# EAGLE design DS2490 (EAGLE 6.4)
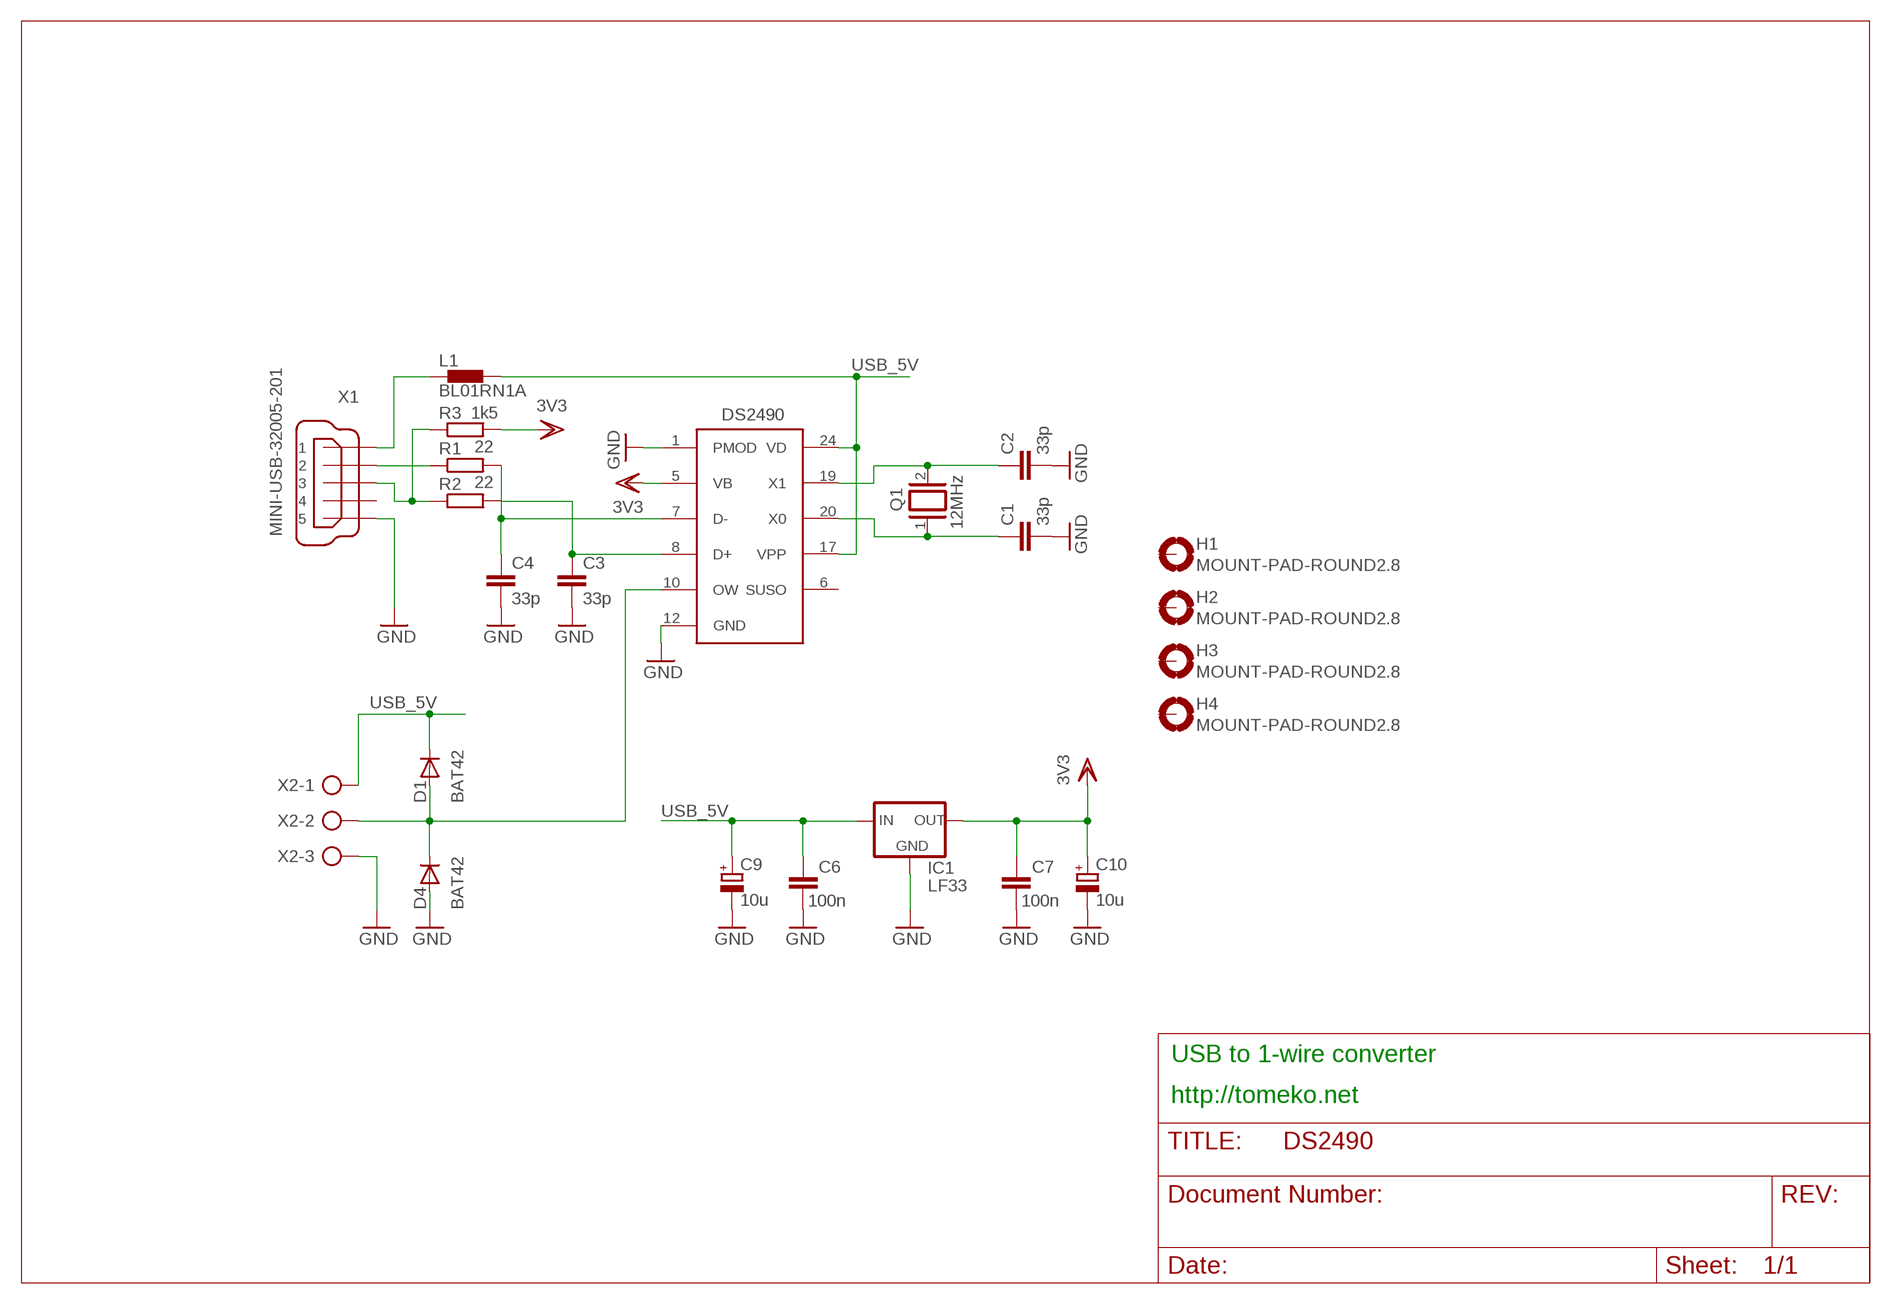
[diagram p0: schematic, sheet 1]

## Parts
C1  33p  C-EUC0805K  [C0805K]
C2  33p  C-EUC0805K  [C0805K]
C3  33p  C-EUC0805K  [C0805K]
C4  33p  C-EUC0805K  [C0805K]
C6  100n  C-EUC0805K  [C0805K]
C7  100n  C-EUC0805K  [C0805K]
C9  10u  CPOL-EUCT3216  [CT3216]
C10  10u  CPOL-EUCT3216  [CT3216]
D1  BAT42  1N4148DO35-7  [DO35-7]
D4  BAT42  1N4148DO35-7  [DO35-7]
H1  MOUNT-PAD-ROUND2.8  [2,8-PAD]
H2  MOUNT-PAD-ROUND2.8  [2,8-PAD]
H3  MOUNT-PAD-ROUND2.8  [2,8-PAD]
H4  MOUNT-PAD-ROUND2.8  [2,8-PAD]
IC1  LF33  LFXXCV  [DPACK_1]
L1  BL01RN1A  [BL01RN1A]
Q1  XTAL/S  [QS]
R1  22  R-EU_R0805  [R0805_40M_SPACE]
R2  22  R-EU_R0805  [R0805_40M_SPACE]
R3  1k5  R-EU_R0805  [R0805_40M_SPACE]
U$1  DS2490  [SO24]
X1  MINI-USB-32005-201  [32005-201]
X2  AK500/3  [AK500/3]

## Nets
ADC_B: D1.A D4.C U$1.10(OW) X2.2
GND: C1.2 C2.2 C3.2 C4.2 C6.1 C7.1 C9.- C10.- D4.A IC1.C(GND) U$1.1(PMOD) U$1.12(GND) X1.5 X2.3
N$1: C2.1 Q1.2 U$1.19(X1)
N$2: R1.1 X1.2
N$3: C1.1 Q1.1 U$1.20(X0)
N$4: L1.1 X1.1
N$5: R2.1 R3.1 X1.3
N$6: C3.1 R2.2 U$1.8(D+)
N$7: C4.1 R1.2 U$1.7(D-)
USB_5V: C6.2 C9.+ D1.C IC1.B(IN) L1.2 U$1.17(VPP) U$1.24(VD) X2.1
VDD: C7.2 C10.+ IC1.E(OUT) R3.2 U$1.5(VB) ; supply symbol labelled 3V3
Unconnected: H1.B2,8(MOUNT) H2.B2,8(MOUNT) H3.B2,8(MOUNT) H4.B2,8(MOUNT) U$1.6(SUSO) X1.4

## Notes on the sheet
- USB to 1-wire converter
- http://tomeko.net

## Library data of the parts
C1-C4 C6 C7 = resistor:C-EU: CAPACITOR, European symbol
C9 C10 = resistor:CPOL-EU: POLARIZED CAPACITOR, European symbol
D1 D4 = diode:1N4148: DIODE
H1-H4 = holes:MOUNT-PAD-ROUND: MOUNTING PAD, round
IC1 = lf33:LFXXCV: VOLTAGE REGULATOR
L1 = inductors:BL0: Noise Suppression Products/EMI Suppression Filters, Lead EMIFIL(R) Inductor Type
Q1 = special:XTAL/S: CRYSTAL; FREQ: 12MHz
R1-R3 = resistor:R-EU_: RESISTOR, European symbol
U$1 = user1wire:DS2490; NM: DS2490
X1 = con-cypressindustries:MINI-USB-: MINI USB-B Conector Source: www.cypressindustries.com; OC_FARNELL: unknown; OC_NEWARK: unknown
X2 = con-ptr500:AK500/3: CONNECTOR; OC_FARNELL: unknown; OC_NEWARK: unknown

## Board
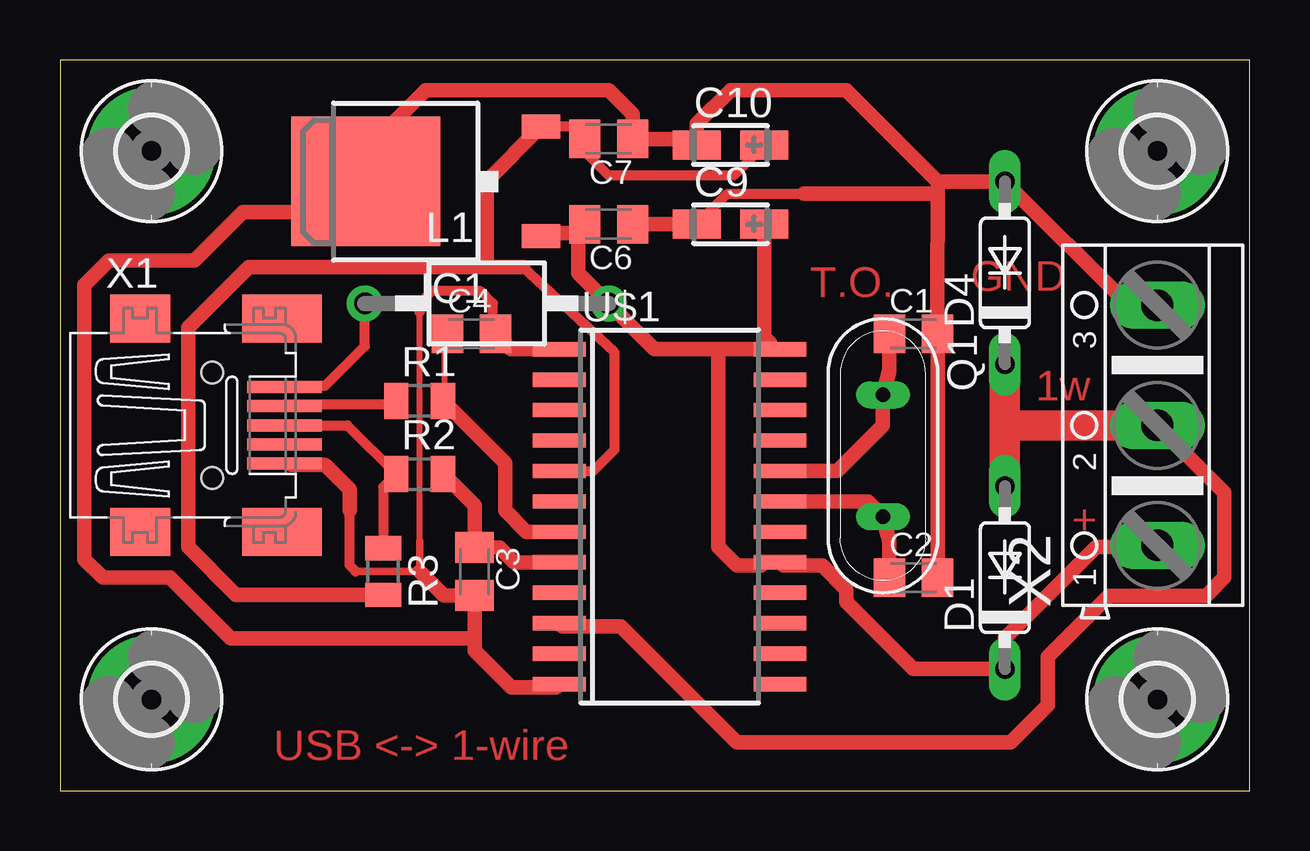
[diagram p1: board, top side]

Size 49.58 x 30.47 mm. Coordinates in mm from the lower left corner, seen from the top.
Outline: 0,0 49.58,0 49.58,30.47 0,30.47 0,0
Copper layers (1*16): Top 0.035mm / dielectric 1.5mm / Bottom 0.035mm
Design rules "default *": minimum track width 10mil, minimum drill 24mil, track to track 10mil, track to pad 9mil, pad to pad 10mil, via to via 10mil, smd to smd 10mil, copper to edge 40mil, drill to drill 8mil, minimum pad ring 10mil, minimum via ring 8mil, stop-mask expansion 4mil, vias tented up to drill 0mil, thermal gap 10mil

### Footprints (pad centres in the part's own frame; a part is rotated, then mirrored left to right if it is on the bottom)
C0805K = smd 1.3 x 1.6: 1 -1,0; 2 1,0
CT3216 = smd 2 x 1.2: + 1.4,0; - -1.4,0
DO35-7 = drill 0.813 long: A 3.81,0; C -3.81,0
2,8-PAD = drill 2.8 pad 5.334: B2,8 0,0
DPACK_1 = smd 1 x 1.6: B -2.28,-4.8; E 2.28,-4.8 | smd 5.4 x 6.2: C 0,2.5
BL01RN1A = drill 0.9 pad 1.5: 1 -5.08,0; 2 5.08,0
QS = drill 0.61 long: 1 -2.54,0; 2 2.54,0
R0805_40M_SPACE = smd 1.016 x 1.5: 1 -0.977,0; 2 0.977,0
SO24 = smd 0.6 x 2.2: 1 -6.985,-4.6; 2 -5.715,-4.6; 3 -4.445,-4.6; 4 -3.175,-4.6; 5 -1.905,-4.6; 6 -0.635,-4.6; 7 0.635,-4.6; 8 1.905,-4.6; 9 3.175,-4.6; 10 4.445,-4.6; 11 5.715,-4.6; 12 6.985,-4.6; 13 6.985,4.6; 14 5.715,4.6; 15 4.445,4.6; 16 3.175,4.6; 17 1.905,4.6; 18 0.635,4.6; 19 -0.635,4.6; 20 -1.905,4.6; 21 -3.175,4.6; 22 -4.445,4.6; 23 -5.715,4.6; 24 -6.985,4.6
32005-201 = smd 3.1 x 0.5: 1 3,1.6; 2 3,0.8; 3 3,0; 4 3,-0.8; 5 3,-1.6 | smd 2.5 x 2: M1 -3,-4.45; M2 -3,4.45 | smd 3.3 x 2: M3 2.9,4.45; M4 2.9,-4.45 | hole 0.9: 0,2.2; 0,-2.2
AK500/3 = drill 1.321 long: 1 -5.004,0; 2 0,0; 3 5.004,0

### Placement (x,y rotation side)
C1  35.56,19.05 0 top
C2  35.56,8.89 0 top
C3  17.27,9.14 270 top
C4  17.14,19.05 0 top
C6  22.86,23.62 180 top
C7  22.86,27.18 180 top
C9  27.94,23.62 0 top
C10  27.94,26.92 0 top
D1  39.37,8.89 90 top
D4  39.37,21.59 90 top
H1  3.81,3.81 0 top
H2  3.81,26.67 0 top
H3  45.72,26.67 0 top
H4  45.72,3.81 0 top
IC1  15.24,25.4 90 top
L1  17.78,20.32 0 top
Q1  34.29,13.97 270 top
R1  14.99,16.26 0 top
R2  14.99,13.21 0 top
R3  13.46,9.14 270 top
U$1  25.4,11.43 270 top
X1  6.35,15.24 0 top
X2  45.72,15.24 90 top

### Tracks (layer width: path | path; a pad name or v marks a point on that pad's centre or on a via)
ADC_B
  Top 0.61: U$1.10 20.93,6.86 23.37,6.86 28.19,2.03 39.62,2.03 41.15,3.56 41.15,5.59 43.69,8.13 47.75,8.13 48.51,8.89 48.51,12.45 X2.2
  Top 1.27: D1.A 39.37,15.24 | X2.2 39.37,15.24 | D4.C 39.37,15.24
GND
  Top 0.254: 20.7,18.41 U$1.1 | 20.83,4.45 U$1.12 | 14.99,10.41 14.99,19.94 | 18.03,19.05 C4.2 | 17.27,8.13 C3.2 | 9.65,13.59 9.4,13.59 X1.5 | 26.16,27.18 26.42,26.92 C10.- | 23.88,27.18 C7.1 | 12.7,25.4 IC1.C
  Top 0.305: 12.32,9.14 14.99,9.14 14.99,10.41
  Top 0.406: 12.06,11.68 12.06,9.4 12.32,9.14 | C9.- 27.81,24.89 30.99,24.89 | 18.03,19.05 18.03,20.32 17.53,20.83 15.49,20.83 14.99,20.32 14.99,19.94
  Top 0.61: C2.2 36.58,10.18 36.58,17.76 C1.2 36.56,20.84 36.58,24.89 | X2.3 44.53,20.24 D4.A 36.58,25.4 | 30.99,24.89 36.58,24.89 | 36.58,25.4 36.58,24.89 | C10.- 26.54,27.81 27.94,29.21 32.77,29.21 36.58,25.4 | 26.16,27.18 C7.1 23.86,28.21 22.86,29.21 15.24,29.21 12.74,26.71 IC1.C | C9.- C6.1 | U$1.12 20.67,4.32 18.8,4.32 17.27,5.84 17.27,6.35 | 17.27,6.35 C3.2 15.99,8.14 14.99,9.14 | 20.7,18.41 18.78,18.41 C4.2 | 9.65,13.59 11.05,13.59 12.06,12.57 12.06,11.68 | 12.7,25.4 11.43,24.13 7.62,24.13 5.59,22.1 2.03,22.1 1.02,21.08 1.02,9.65 1.78,8.89 4.57,8.89 7.11,6.35 17.27,6.35
N$1
  Top 0.61: U$1.19 33.66,12.06 Q1.2 34.56,10.43 C2.1
N$2
  Top 0.254: 9.4,16.13 X1.2
  Top 0.406: 9.4,16.13 13.88,16.13 R1.1
N$3
  Top 0.61: U$1.20 32.38,13.34 34.29,15.24 Q1.1 34.56,17.51 C1.1
N$4
  Top 0.254: 12.7,19.94 L1.1 | 9.65,16.89 9.4,16.89 X1.1
  Top 0.406: 9.65,16.89 11.05,16.89 12.7,18.54 L1.1
N$5
  Top 0.406: X1.3 11.98,15.24 R2.1 13.46,12.66 R3.1
N$6
  Top 0.254: 16,13.21 R2.2 | 17.27,10.16 C3.1 17.27,10.03
  Top 0.61: U$1.8 18.92,9.53 18.3,10.14 C3.1 | 17.27,10.16 17.27,11.9 R2.2
N$7
  Top 0.254: C4.1 16,18.92 16,16.26 R1.2
  Top 0.61: U$1.7 19.43,10.79 18.54,11.68 18.54,13.68 R1.2
USB_5V
  Top 0.254: 45.72,10.16 X2.1 | 21.46,23.24 21.84,23.62 C6.2 21.59,23.24 | 20.07,23.24 IC1.B | 29.34,9.53 U$1.17 | 29.59,18.67 U$1.24
  Top 0.61: 45.72,10.16 43.18,10.16 39.37,6.35 D1.C 35.56,5.08 32.77,7.87 32.77,8.38 31.75,9.4 30.13,9.4 U$1.17 | 20.07,23.24 21.46,23.24 | 21.59,23.24 21.59,21.59 L1.2 24.77,18.41 27.43,18.41 | 27.43,18.41 U$1.24 | 29.59,18.67 29.34,18.92 C9.+ | 29.34,9.53 29.21,9.4 28.19,9.4 27.43,10.16 27.43,18.41
VDD
  Top 0.254: 13.46,8.26 R3.2 | 21.84,27.18 C7.2 | 20.07,27.56 IC1.E
  Top 0.406: C10.+ 28.07,25.65 22.86,25.65 21.86,26.65 C7.2 21.36,27.68 IC1.E | U$1.5 22.23,13.34 23.11,14.22 23.11,18.29 19.3,21.84
  Top 0.61: 17.78,21.84 7.87,21.84 5.33,19.3 5.33,10.16 7.33,8.17 R3.2 | 19.3,21.84 17.78,21.84 | 17.78,21.84 17.78,25.42 IC1.E

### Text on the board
Top: GND | T.O. | 1w | + | USB <-> 1-wire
